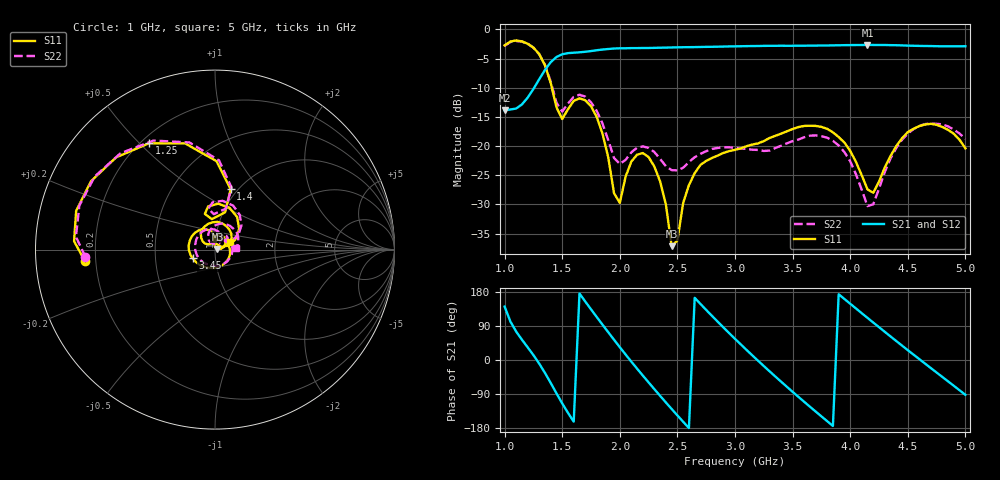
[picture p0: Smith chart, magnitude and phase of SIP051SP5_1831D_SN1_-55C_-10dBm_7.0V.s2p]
# GHz  S  dB  R  50
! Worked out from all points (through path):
!   81 points, 1 GHz to 5 GHz, reference 50 ohm
!   highest |S21| = -2.66 dB at 4.15 GHz (marker M1); lowest = -13.9 dB at 1 GHz (marker M2)
!   lowest |S11| = -37.1 dB at 2.45 GHz (marker M3), VSWR 1.03, Z = 51.3 + j0.411 ohm
!   |S11| at or under -10 dB: 1.41 GHz to end of sweep
!   |S22| runs from -30.3 to -2.0 dB; largest |S21 - S12| = 0.002
!   S11 on the Smith chart (normalised r, x): 1 GHz: 0.16, -0.04; 1.25 GHz: 0.23, +0.53; 1.4 GHz: 0.93, +0.71; 3.45 GHz: 0.77, -0.08; 5 GHz: 1.18, +0.10
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1  -2.75 -175.1  -13.86 141.0  -13.86 141.1  -2.82 -176.8
1.25  -3.13 121.8  -10.22 13.0  -10.23 13.0  -3.13 119.4
1.4  -9.18 75.4  -5.63 -60.4  -5.64 -60.4  -8.94 75.0
1.5  -15.37 95.8  -4.27 -114.4  -4.26 -114.5  -14.09 92.0
1.7  -12.15 71.2  -3.84 154.4  -3.85 154.4  -11.53 67.5
1.85  -17.88 26.6  -3.46 93.2  -3.46 93.2  -16.14 32.7
1.95  -28.09 24.3  -3.28 53.4  -3.30 53.4  -22.03 34.7
2.05  -25.26 95.3  -3.24 14.6  -3.25 14.6  -22.36 62.0
2.2  -21.20 58.4  -3.20 -41.2  -3.22 -41.1  -20.05 49.9
2.35  -26.07 15.6  -3.15 -94.6  -3.15 -94.6  -22.20 33.7
2.45  -37.15 16.8  -3.10 -129.2  -3.11 -129.2  -24.12 37.7
2.65  -24.64 70.4  -3.04 164.1  -3.03 164.2  -21.91 43.8
2.85  -21.62 0.8  -2.97 101.1  -2.97 101.0  -20.32 14.5
3  -20.65 -49.0  -2.92 55.8  -2.91 55.9  -20.28 -16.8
3.2  -19.55 -104.9  -2.86 -1.9  -2.85 -1.9  -20.66 -74.8
3.45  -17.47 -158.8  -2.82 -70.6  -2.81 -70.6  -19.54 -162.1
3.7  -16.54 150.3  -2.79 -135.9  -2.79 -135.9  -18.18 124.6
3.9  -18.45 111.7  -2.73 173.5  -2.73 173.5  -19.89 78.5
4.15  -27.41 105.0  -2.66 111.2  -2.67 111.2  -30.28 72.8
4.35  -21.70 146.2  -2.71 62.2  -2.72 62.2  -22.12 119.3
4.65  -16.31 94.4  -2.86 -9.4  -2.86 -9.5  -16.24 67.4
5  -20.39 25.9  -2.89 -91.9  -2.90 -91.9  -18.78 3.2
